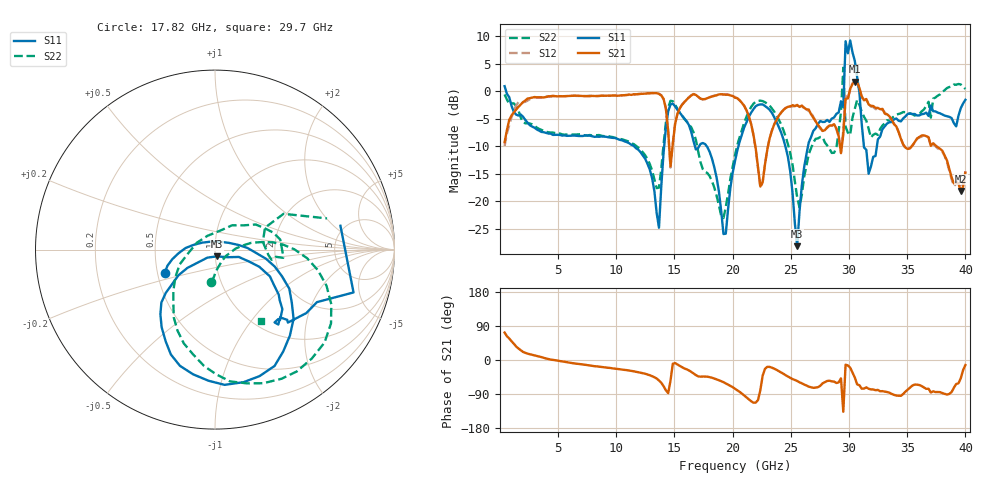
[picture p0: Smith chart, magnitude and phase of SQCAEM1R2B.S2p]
! Network Analyzer HP8722ES.07.66: Jul 25, 2000 Serial No. US39175408
! 26 Oct 2004  10:46:45
! Frequency  S11  S21  S12  S22
# HZ  S  DB R  50
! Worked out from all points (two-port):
!   201 points, 400 MHz to 40 GHz, reference 50 ohm
!   highest |S21| = 1.70 dB at 30.5 GHz (marker M1); lowest = -18.2 dB at 39.6 GHz (marker M2)
!   |S21| within 3 dB of the highest: 2.562 GHz to 14.02 GHz (11.46 GHz wide, 138 % of centre); 17.82 GHz to 20.4 GHz (2.579 GHz wide, 13.5 % of centre)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
!   lowest |S11| = -28.2 dB at 25.55 GHz (marker M3), VSWR 1.08, Z = 50.9 - j3.83 ohm
!   |S11| at or under -10 dB: 11.5 GHz to 14.11 GHz (2.612 GHz wide, 20.4 % of centre); 17.76 GHz to 20.5 GHz (2.743 GHz wide, 14.3 % of centre); 24.52 GHz to 26.48 GHz (1.955 GHz wide, 7.67 % of centre)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
!   |S22| runs from -23.1 to 4.2 dB; largest |S21 - S12| = 0.18
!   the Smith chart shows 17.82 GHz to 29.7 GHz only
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4e8  0.88 -18.5  -9.31 72.4  -10.00 77.3  -0.62 -10.9
7.132e9  -8.18 -105.0  -0.91 -11.8  -0.93 -12.4  -7.99 -100.5
1.3666e10  -24.85 93.1  -0.51 -54.1  -0.51 -53.9  -17.56 -40.9
1.4656e10  -2.44 -58.2  -13.70 -54.8  -13.92 -53.0  -1.78 -50.5
1.624e10  -6.19 -140.3  -1.17 -27.6  -1.11 -27.5  -6.04 -101.9
1.921e10  -26.00 117.7  -0.64 -58.5  -0.58 -58.9  -23.09 -31.2
2.02e10  -12.73 -4.8  -1.21 -76.0  -1.08 -75.4  -11.63 9.2
2.2378e10  -2.43 -77.9  -17.36 -79.6  -17.54 -77.4  -1.75 -56.1
2.3368e10  -3.96 -112.8  -7.25 -20.2  -7.16 -19.6  -3.16 -89.4
2.5546e10  -28.20 -74.9  -2.52 -55.5  -2.66 -55.1  -19.36 158.8
2.6932e10  -7.24 -35.2  -4.86 -73.5  -4.70 -73.2  -9.37 15.9
2.9308e10  -1.85 -17.2  -11.29 -48.5  -11.20 -47.4  -3.77 15.6
2.9506e10  -2.96 10.8  -7.90 -136.5  -7.16 -117.8  4.25 40.9
2.9704e10  9.05 -3.6  -1.38 -12.3  -0.86 -1.3  -6.50 -56.9
2.9902e10  6.86 -61.7  -1.35 -14.5  -1.40 -13.3  -7.57 8.6
3.01e10  9.19 -77.1  0.37 -20.2  0.36 -19.4  -8.00 16.6
3.0496e10  5.48 -101.1  1.70 -46.2  1.91 -45.3  -3.23 -4.4
3.0694e10  2.59 50.2  1.63 -64.2  1.61 -63.2  -1.64 161.0
3.1486e10  -10.68 -105.3  -1.45 -72.2  -1.61 -72.8  -5.40 -36.6
3.3466e10  -5.68 -31.5  -4.59 -86.2  -4.85 -85.9  -5.34 -4.7
3.9604e10  -3.12 -55.6  -18.18 -48.1  -17.62 -42.1  1.19 -4.1
4e10  -1.60 -59.6  -14.84 -13.2  -14.60 -12.4  0.37 -15.8
